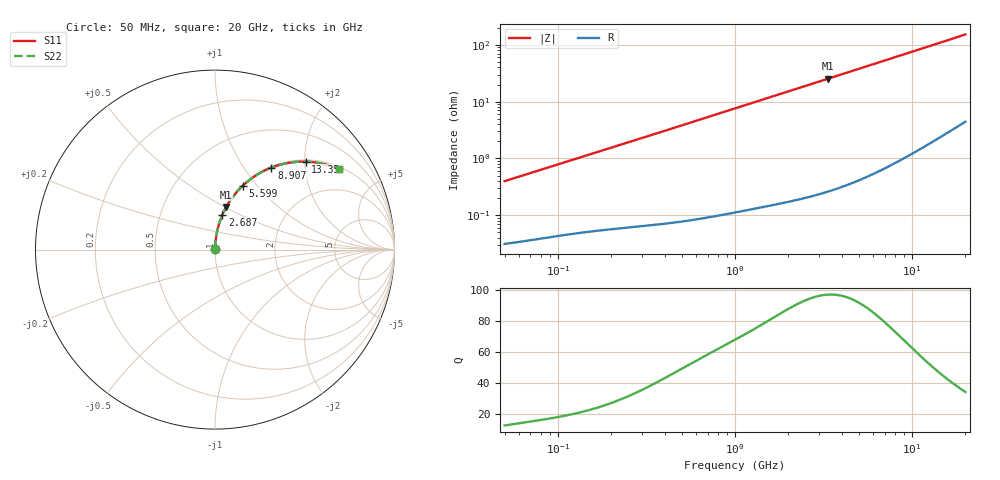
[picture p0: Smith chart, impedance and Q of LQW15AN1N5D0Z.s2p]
!Murata Part Number: LQW15AN1N5D0Z
!These Parameters are Measured in Series Mode Connection
!  o--[Z]--o
!Port1  Port2
!  o-------o
!Freq. Start=50[MHz] Stop=20[GHz], 401[Steps]
# Hz S RI R 50
!Freq.(Hz) S11(Real) S11(Imag) S21(Real) S21(Imag) S12(Real) S12(Imag) S22(Real) S22(Imag)
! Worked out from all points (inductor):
!   401 points, 50 MHz to 20 GHz, reference 50 ohm
!   read as one part in series: L = 1.26 nH near 51.52 MHz
!   highest Q = 97.1 at 3.364 GHz (marker M1), where L = 1.2 nH
!   S11 on the Smith chart (normalised r, x): 50 MHz: 1.00, +0.01; 2.687 GHz: 1.00, +0.41; 5.599 GHz: 1.01, +0.85; 8.907 GHz: 1.02, +1.35; 13.35 GHz: 1.04, +2.02; 20 GHz: 1.09, +3.04
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5e7  0.000328 0.00396  0.9997 -0.00396  0.9997 -0.00396  0.000328 0.00396
5.152053e7  0.000333 0.00408  0.9997 -0.00408  0.9997 -0.00408  0.000333 0.00408
1.364002e8  0.000606 0.0106  0.9994 -0.0106  0.9994 -0.0106  0.000606 0.0106
3.721004e8  0.00149 0.0284  0.9985 -0.0284  0.9985 -0.0284  0.00149 0.0284
6.380365e8  0.00321 0.0484  0.9968 -0.0484  0.9968 -0.0484  0.00321 0.0484
1e9  0.00682 0.0753  0.9932 -0.0753  0.9932 -0.0753  0.00682 0.0753
1.309461e9  0.011 0.098  0.989 -0.098  0.989 -0.098  0.011 0.098
1.689197e9  0.0175 0.1254  0.9825 -0.1254  0.9825 -0.1254  0.0175 0.1254
2.146657e9  0.0273 0.1575  0.9727 -0.1575  0.9727 -0.1575  0.0273 0.1575
2.687447e9  0.0415 0.1942  0.9585 -0.1942  0.9585 -0.1942  0.0415 0.1942
2.728004e9  0.0426 0.1968  0.9574 -0.1968  0.9574 -0.1968  0.0426 0.1968
3.364474e9  0.0628 0.2375  0.9372 -0.2375  0.9372 -0.2375  0.0628 0.2375
4.405649e9  0.1021 0.2975  0.8979 -0.2975  0.8979 -0.2975  0.1021 0.2975
5.598765e9  0.1543 0.3557  0.8457 -0.3557  0.8457 -0.3557  0.1543 0.3557
6.503449e9  0.1971 0.3918  0.8029 -0.3918  0.8029 -0.3918  0.1971 0.3918
7.442007e9  0.2429 0.4223  0.7571 -0.4223  0.7571 -0.4223  0.2429 0.4223
8.907419e9  0.3142 0.4569  0.6858 -0.4569  0.6858 -0.4569  0.3142 0.4569
1.098561e10  0.4098 0.4833  0.5902 -0.4833  0.5902 -0.4833  0.4098 0.4833
1.334722e10  0.5051 0.49  0.4949 -0.49  0.4949 -0.49  0.5051 0.49
1.597544e10  0.5925 0.4797  0.4075 -0.4797  0.4075 -0.4797  0.5925 0.4797
1.912117e10  0.6741 0.4549  0.3259 -0.4549  0.3259 -0.4549  0.6741 0.4549
2e10  0.6931 0.4469  0.3069 -0.4469  0.3069 -0.4469  0.6931 0.4469
